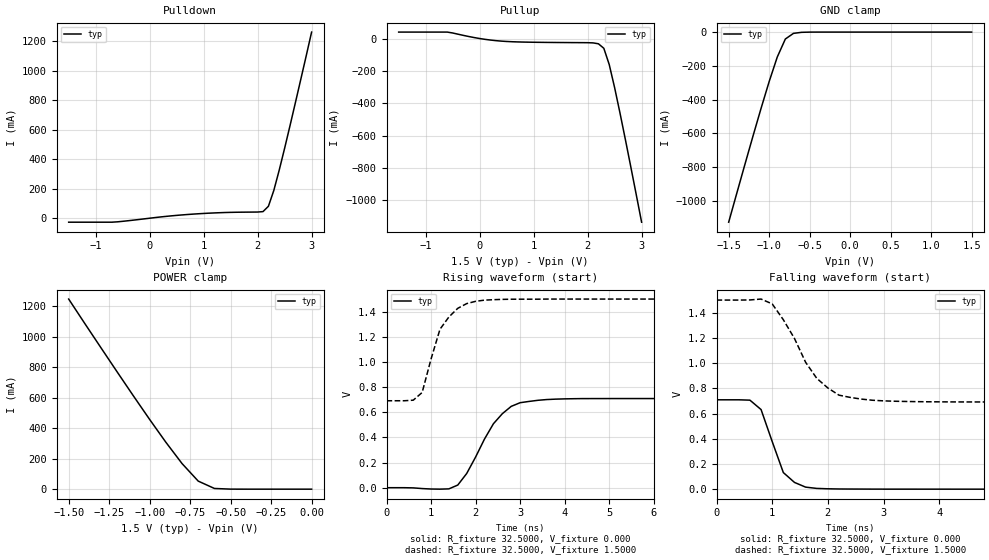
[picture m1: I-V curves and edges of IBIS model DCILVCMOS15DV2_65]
| / 7\'7
| \ \   Xilinx Inc.
| / /
| \_\/.\   IBIS Model for Virtex-II
[IBIS ver]   2.1
[File name]   dci1565d.ibs
[File Rev]   1.1
[Date]   Aug. 1, 2001
[Source]   Hspice simulations (08-01: TT, SS, FF)
[Notes]   Xilinx IBIS model for LVDCI 1.5V 32.5 ohms (65/2) driver.
[Disclaimer] The data in this model is derived from SPICE simulations using
   modeling information extracted from the target process. While
   a great deal of care has been taken to provide information
   that is accurate, this model is considered preliminary as it
   has not been verified by actual silicon measurement. Treat the
   data in this model as preliminary until actual silicon
   verification is performed.
[Copyright]   Copyright 2001, Xilinx Inc., All rights reserved
|   Component Virtex_II
[Component]   Virtex_II
[Manufacturer]   Xilinx Inc.
[Package]
| variable   typ   min   max
R_pkg   0.1   NA   NA
L_pkg   0.8nH   NA   NA
C_pkg   0.5pF   NA   NA
[Pin]  signal_name   model_name   R_pin   L_pin   C_pin
io   DCILVCMOS15DV2_65   DCILVCMOS15DV2_65
| ins  insig   inp
| ens  ensig   inp
PGND   GND   GND
VCCO   VCCO   POWER
| Models and submodels in the file (1): DCILVCMOS15DV2_65 (I/O)
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|   Model DCILVCMOS15DV2_65
[Model]   DCILVCMOS15DV2_65
Model_type   I/O
Polarity   Non-Inverting
Enable   Active-Low
Vinh = 1.05V
Vinl = 0.3V
Vmeas =   0.7300V
Cref =  35.0000pF
Rref =   1.0000M
Vref =  0.000V
C_comp   7.0000pF   NA   NA
[Temperature Range]   25.0000   NA   NA
[Voltage Range]   1.5000V   NA   NA
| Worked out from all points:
|   slope of the pulldown table from 0 to 0.225 V, typ, clamps not added: 23.9 ohm
|   slope of the pullup table from 0 to 0.225 V, typ, clamps not added: 21.7 ohm
|   GND clamp passes 1 mA (typ) near -0.57 V on its own axis
|   POWER clamp passes 1 mA (typ) near -0.52 V on its own axis
|   rising waveform, R_fixture 32.5000, V_fixture 0.000: 20-80 % time 703ps typ, NA min, NA max; typ from 0 V to 0.709 V
|   rising waveform, R_fixture 32.5000, V_fixture 1.5000: 20-80 % time 489ps typ, NA min, NA max; typ from 0.691 V to 1.5 V
|   falling waveform, R_fixture 32.5000, V_fixture 0.000: 20-80 % time 341ps typ, NA min, NA max; typ from 0.709 V to 0 V
|   falling waveform, R_fixture 32.5000, V_fixture 1.5000: 20-80 % time 660ps typ, NA min, NA max; typ from 1.5 V to 0.692 V
[Pulldown]
| voltage   I(typ)   I(min)   I(max)
-1.5V     -26.93mA   NA         NA
-700mV    -26.93mA   NA         NA
800mV     27.71mA    NA         NA
2.1V      44.78mA    NA         NA
2.2V      80.94mA    NA         NA
2.3V      188.1mA    NA         NA
2.4V      325.6mA    NA         NA
2.5V      473.6mA    NA         NA
2.7V      783.3mA    NA         NA
3V        1.261A     NA         NA
[Pullup]
| voltage   I(typ)   I(min)   I(max)
-1.5V     39.79mA    NA         NA
-600mV    39.79mA    NA         NA
0V        -9.4nA     NA         NA
500mV     -18.25mA   NA         NA
2V        -25.82mA   NA         NA
2.2V      -32.54mA   NA         NA
2.3V      -60.37mA   NA         NA
2.4V      -160.6mA   NA         NA
2.5V      -303.6mA   NA         NA
2.6V      -461.4mA   NA         NA
2.8V      -793.9mA   NA         NA
3V        -1.136A    NA         NA
[GND_clamp]
| voltage   I(typ)   I(min)   I(max)
-1.5V     -1.127A    NA         NA
-1.2V     -617mA     NA         NA
-1V       -293.4mA   NA         NA
-900mV    -148mA     NA         NA
-800mV    -41mA      NA         NA
-700mV    -7.588mA   NA         NA
-600mV    -1.413mA   NA         NA
1.5V      218.4nA    NA         NA
[POWER_clamp]
| voltage   I(typ)   I(min)   I(max)
-1.5V     1.246A     NA         NA
-1.1V     610.9mA    NA         NA
-900mV    307.7mA    NA         NA
-800mV    167.8mA    NA         NA
-700mV    52.78mA    NA         NA
-600mV    4.607mA    NA         NA
0V        218.4nA    NA         NA
[Ramp]
| variable   typ   min   max
dV/dt_r   0.4253/0.6878n   NA   NA
dV/dt_f   0.4851/0.6071n   NA   NA
R_load = 32.5000
[Rising Waveform]
R_fixture = 32.5000
V_fixture = 0.000
| time   V(typ)   V(min)   V(max)
0s        4.725uV    NA         NA
1.4ns     -9.368mV   NA         NA
1.6ns     21.11mV    NA         NA
1.8ns     113mV      NA         NA
2.4ns     508.5mV    NA         NA
2.6ns     588.4mV    NA         NA
2.8ns     646.8mV    NA         NA
3ns       675.9mV    NA         NA
4.2ns     707.6mV    NA         NA
10ns      708.9mV    NA         NA
[Rising Waveform]
R_fixture = 32.5000
V_fixture = 1.5000
V_fixture_min = 1.4000
V_fixture_max = 1.6000
| time   V(typ)   V(min)   V(max)
0s        691.4mV    NA         NA
600ps     695.9mV    NA         NA
800ps     757.2mV    NA         NA
1ns       1.024V     NA         NA
1.2ns     1.26V      NA         NA
1.4ns     1.357V     NA         NA
1.6ns     1.427V     NA         NA
2ns       1.482V     NA         NA
2.8ns     1.499V     NA         NA
10ns      1.5V       NA         NA
[Falling Waveform]
R_fixture = 32.5000
V_fixture = 0.000
| time   V(typ)   V(min)   V(max)
0s        708.9mV    NA         NA
600ps     706mV      NA         NA
800ps     631.5mV    NA         NA
1ns       377.8mV    NA         NA
1.2ns     131.7mV    NA         NA
1.4ns     53.57mV    NA         NA
1.6ns     16.17mV    NA         NA
1.8ns     5.958mV    NA         NA
2.4ns     1.012mV    NA         NA
10ns      -14.79uV   NA         NA
[Falling Waveform]
R_fixture = 32.5000
V_fixture = 1.5000
V_fixture_min = 1.4000
V_fixture_max = 1.6000
| time   V(typ)   V(min)   V(max)
0s        1.5V       NA         NA
800ps     1.508V     NA         NA
1ns       1.47V      NA         NA
1.2ns     1.344V     NA         NA
1.6ns     1.007V     NA         NA
1.8ns     879.3mV    NA         NA
2.2ns     745.6mV    NA         NA
2.4ns     728mV      NA         NA
3.8ns     693.2mV    NA         NA
10ns      691.5mV    NA         NA
